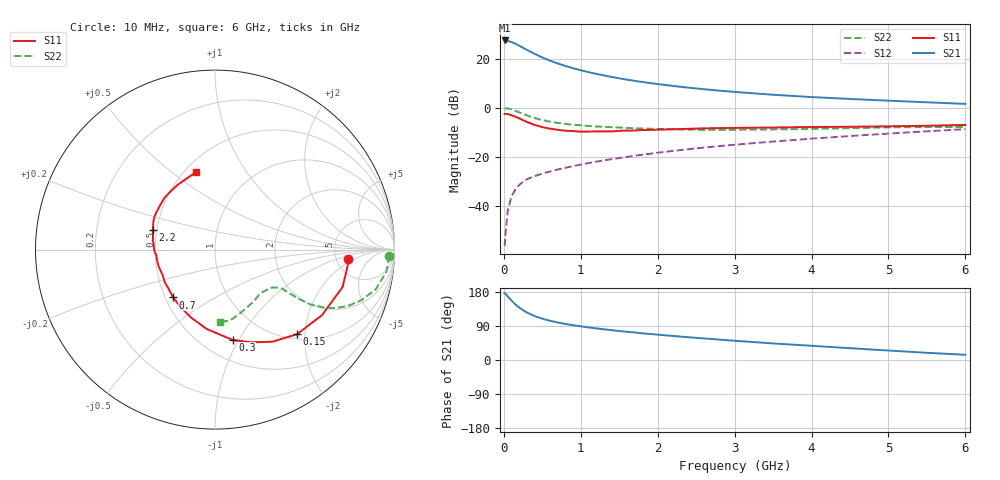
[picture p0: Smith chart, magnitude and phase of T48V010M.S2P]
! Infineon Technologies  Discrete & RF Semiconductors
! BFR182T
! Si NPN RF Bipolar Junction Transistor in SC75
! VCE = 8 V  IC = 10 mA
! Common Emitter S-Parameters:  October  1999
# GHz  S  MA  R  50
!  f  S11  S21  S12  S22
! GHz  MAG  ANG  MAG  ANG  MAG  ANG  MAG  ANG
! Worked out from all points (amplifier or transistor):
!   36 points, 10 MHz to 6 GHz, reference 50 ohm
!   highest |S21| = 27.4 dB at 10 MHz (marker M1)
!   |S21| within 3 dB of that: start of sweep to 250.9 MHz
!   unconditionally stable (mu >= 1): 1.109 GHz to 3.992 GHz
!   at 250 MHz: K = 0.42, MSG = 27.3 dB, |S12| = -30.2 dB
!   at 1.4 GHz: K = 1.05, MAG = 15.4 dB, |S12| = -21.0 dB
!   at 6 GHz: K = 0.86, MSG = 5.2 dB, |S12| = -8.8 dB
!   lowest NFmin = 1.50 dB at 450 MHz
!   S11 on the Smith chart (normalised r, x): 10 MHz: 6.38, -1.55; 150 MHz: 1.10, -1.82; 300 MHz: 0.69, -0.94; 700 MHz: 0.55, -0.34; 2.2 GHz: 0.48, +0.12; 6 GHz: 0.57, +0.62
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0.01  0.7425 -4.2  23.46 176.1  0.0015 77.8  0.9721 -2.1
0.02  0.7475 -5.1  23.19 174.9  0.0025 94.2  0.9702 -2.8
0.05  0.7409 -16.3  22.99 167.7  0.0078 85.7  0.9633 -7.3
0.1  0.6996 -31.4  21.7 156.9  0.0155 76.2  0.9227 -13.9
0.15  0.6565 -45.9  20.13 146.7  0.0216 69.3  0.862 -19.1
0.2  0.6051 -58.0  18.38 138.4  0.0267 67.4  0.8031 -23.1
0.25  0.5539 -68.9  16.64 131.3  0.0308 63.1  0.7446 -25.9
0.3  0.5127 -79.0  15.06 125.3  0.0347 61.7  0.6958 -27.8
0.4  0.4448 -95.9  12.51 115.8  0.0402 58.6  0.6139 -29.9
0.5  0.4018 -109.2  10.58 109.0  0.0452 59.2  0.5591 -30.3
0.6  0.3734 -121.1  9.094 103.5  0.05 58.8  0.5192 -30.5
0.7  0.3539 -131.1  7.985 99.0  0.0549 60.0  0.4884 -30.4
0.9  0.3331 -147.4  6.372 91.8  0.0642 61.4  0.4481 -30.3
1.1  0.3258 -160.4  5.304 85.9  0.0742 62.7  0.4246 -30.6
1.4  0.3283 -174.3  4.231 78.8  0.089 64.2  0.4007 -32.0
1.6  0.3409 177.9  3.731 74.4  0.0991 64.8  0.3864 -33.0
2.2  0.3632 162.6  2.772 63.4  0.1314 65.1  0.3632 -38.7
2.8  0.3833 151.5  2.228 53.9  0.1641 64.1  0.3515 -45.7
3.5  0.3934 140.7  1.833 43.7  0.2038 62.2  0.3612 -54.7
4.5  0.4075 127.5  1.505 31.2  0.2639 58.0  0.3822 -68.8
5.5  0.4274 111.1  1.286 19.0  0.3299 52.9  0.4031 -80.8
6  0.4454 103.4  1.195 13.8  0.3644 49.5  0.4042 -85.7
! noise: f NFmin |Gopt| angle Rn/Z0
0.45  1.5  0.26  43  0.28
0.9  1.6  0.24  87  0.22
1.8  2.1  0.2  170  0.2
